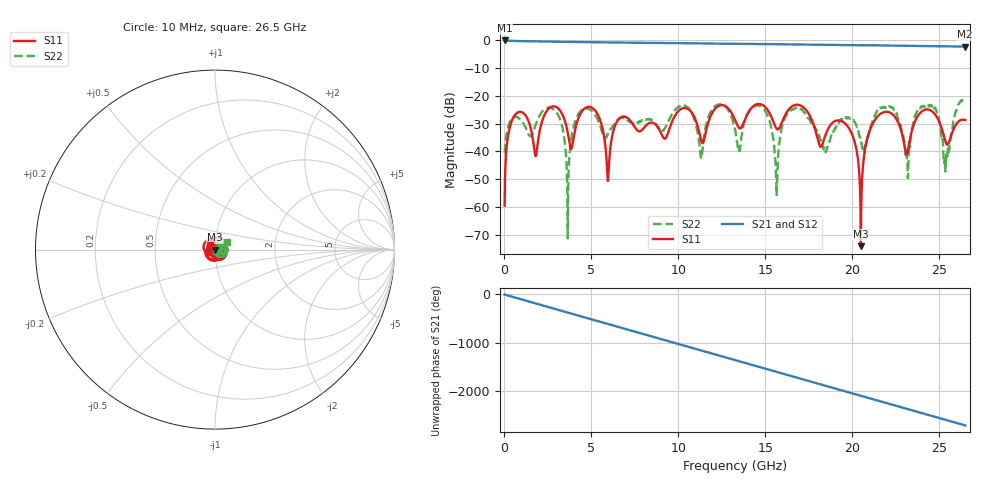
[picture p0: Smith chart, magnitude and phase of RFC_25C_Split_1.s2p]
!Keysight Technologies,N5245B,MY55451909,A.13.80.08
!Automatic Fixture Removal (AFR)
!Date: Thursday, August 27, 2020, 03:53:06
!S2P File: Measurements: S11,S21,S12,S22:
# MHz S  RI  R 50
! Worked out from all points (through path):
!   2650 points, 10 MHz to 26.5 GHz, reference 50 ohm
!   highest |S21| = 0.00 dB at 10 MHz (marker M1); lowest = -2.2 dB at 26.47 GHz (marker M2)
!   group delay of S21, straight-line fit = 284 ps
!   lowest |S11| = -74.2 dB at 20.49 GHz (marker M3), VSWR 1.00, Z = 50 + j0.0195 ohm
!   |S11| at or under -10 dB: start of sweep to end of sweep
!   |S22| runs from -71.4 to -21.5 dB; largest |S21 - S12| = 1.5e-15
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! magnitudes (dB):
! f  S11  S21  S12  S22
! 10 MHz  -59.6  0.0  0.0  -40.5
! 690 MHz  -26.3  -0.2  -0.2  -27.5
! 1.79 GHz  -41.8  -0.3  -0.3  -30.5
! 2.9 GHz  -23.8  -0.5  -0.5  -25.3
! 3.64 GHz  -33.2  -0.5  -0.5  -71.4
! 4.43 GHz  -25.8  -0.6  -0.6  -25.1
! 5.95 GHz  -50.7  -0.7  -0.7  -33.6
! 6.67 GHz  -27.8  -0.8  -0.8  -28.0
! 8.84 GHz  -31.5  -0.9  -0.9  -31.5
! 13.26 GHz  -28.7  -1.2  -1.2  -32.3
! 14.79 GHz  -23.1  -1.3  -1.3  -24.0
! 15.64 GHz  -31.8  -1.4  -1.4  -53.3
! 16.27 GHz  -25.5  -1.4  -1.4  -26.3
! 17.67 GHz  -28.7  -1.5  -1.5  -29.8
! 19.73 GHz  -31.0  -1.7  -1.7  -28.0
! 20.49 GHz  -74.2  -1.7  -1.7  -35.6
! 22.09 GHz  -25.8  -1.8  -1.8  -24.0
! 23.14 GHz  -40.9  -1.9  -1.9  -42.5
! 24.67 GHz  -26.0  -2.1  -2.1  -23.9
! 25.36 GHz  -36.5  -2.1  -2.1  -44.9
! 26.47 GHz  -28.7  -2.2  -2.2  -22.0
! 26.5 GHz  -28.7  -2.2  -2.2  -22.1
